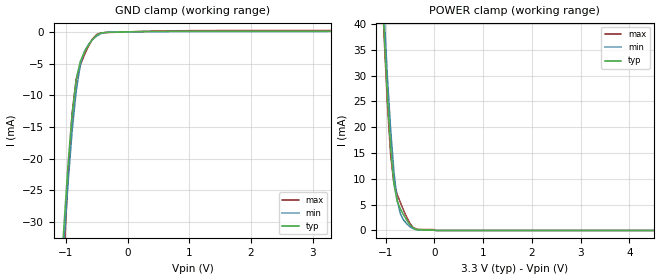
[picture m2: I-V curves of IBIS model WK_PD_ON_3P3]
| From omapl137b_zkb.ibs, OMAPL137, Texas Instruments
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|   Model Cell WK_PD_ON_3P3
|WK_PD_ON_3P3
[Model]   WK_PD_ON_3P3
Model_type   Input
Polarity   Non-Inverting
Vinl =  0.8
Vinh =  2
C_comp   1.652921p   1.424215p   1.79759p
[Model Spec]
Vinl   0.8   0.8   0.8
Vinh   2   2   2
[Temperature Range]   25   125   -40
[Voltage Range]   3.3   2.97   3.63
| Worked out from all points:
|   GND clamp passes 1 mA (typ) near -0.55 V on its own axis
|   POWER clamp passes 1 mA (typ) near -0.49 V on its own axis
| Nom Voltages:
|   VDD=1, VDDS=3.3, VSS=0, VSSS=0
| Min Voltages:
|   VDD=0.99, VDDS=2.97, VSS=0, VSSS=0
| Max Voltages:
|   VDD=1.21, VDDS=3.63, VSS=0, VSSS=0
[POWER_clamp]
|   voltage   I(typ)   I(min)   I(max)
-3.3V     637.1mA    797mA      659.4mA
-1.1V     52.46mA    55.13mA    52.56mA
-1.033V   38.33mA    41.73mA    37.5mA
-966.7mV  25.97mA    29.78mA    24.52mA
-900mV    15.97mA    19.57mA    14.64mA
-833.3mV  9.03mA     11.42mA    9.195mA
-766.7mV  5.685mA    5.91mA     7.02mA
-700mV    4.17mA     3.207mA    5.404mA
-566.7mV  1.964mA    1.272mA    2.49mA
-433.3mV  458.8uA    327uA      539.6uA
33.33mV   0A         0A         0A
6.6V      0A         0A         0A
[GND_clamp]
|   voltage   I(typ)   I(min)   I(max)
-3.3V     -540.5mA   -632.1mA   -650.1mA
-1.1V     -42.2mA    -44.78mA   -50.38mA
-1.033V   -30.95mA   -33.91mA   -36.07mA
-966.7mV  -21.15mA   -24.12mA   -23.18mA
-900mV    -13.09mA   -15.79mA   -13.02mA
-833.3mV  -7.494mA   -9.38mA    -7.574mA
-766.7mV  -4.674mA   -5.239mA   -5.263mA
-700mV    -3.206mA   -3.097mA   -3.638mA
-566.7mV  -1.168mA   -1.217mA   -1.083mA
-500mV    -516.2uA   -650.4uA   -412.9uA
-233.3mV  -47.78uA   -32.35uA   -71.2uA
3.3V      96.87uA    93.84uA    209.4uA
